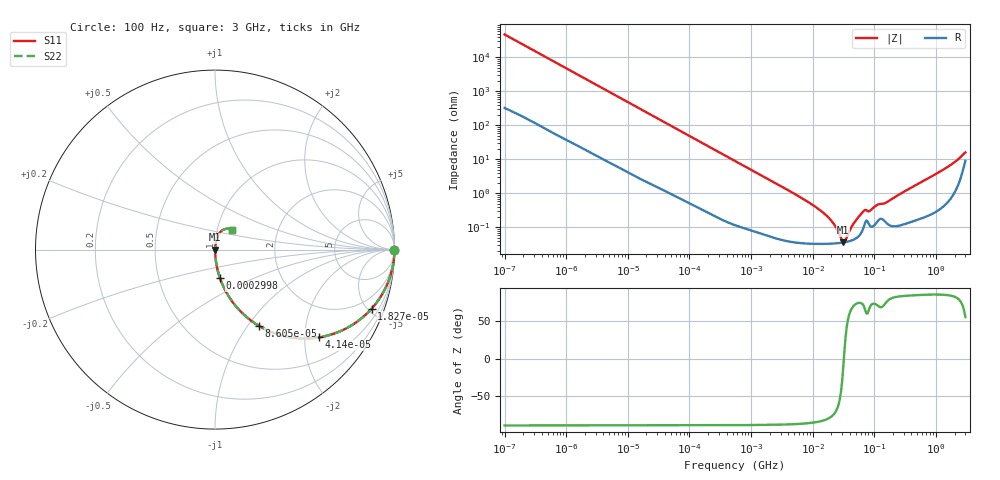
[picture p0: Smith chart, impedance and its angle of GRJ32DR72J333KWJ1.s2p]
!Murata Part Number: GRJ32DR72J333KWJ1
!These Parameters are Measured in Series Mode Connection
!Data Generated on Jun 19, 2026
!  o--ll--o
!Port1  Port2
!  o------o
!Operation Temp=25[degC], DC Bias Voltage=0[V]
!Freq. Start=100[Hz] Stop=3[GHz] 401[Steps]
# Hz S RI R 50
!Freq.(Hz) S11(Real) S11(Imag) S21(Real) S21(Imag) S12(Real) S12(Imag) S22(Real) S22(Imag)
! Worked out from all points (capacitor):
!   401 points, 100 Hz to 3 GHz, reference 50 ohm
!   read as one part in series: C = 33.7 nF near 109 Hz
!   lowest |Z| = 36.6 mohm at 31.31 MHz (marker M1)
!   series resonance near 32.03 MHz, so ESL is about 730 pH
!   S11 on the Smith chart (normalised r, x): 100 Hz: open; 18.27 kHz: 1.05, -5.30; 41.4 kHz: 1.02, -2.35; 86.05 kHz: 1.01, -1.14; 299.8 kHz: 1.00, -0.33; 3 GHz: 1.18, +0.26
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100  1 -0.00212  1.91e-05 0.00212  1.91e-05 0.00212  1 -0.00212
1788  0.9983 -0.0373  0.0017 0.0373  0.0017 0.0373  0.9983 -0.0373
6504  0.981 -0.1323  0.019 0.1323  0.019 0.1323  0.981 -0.1323
18274  0.8732 -0.3284  0.1268 0.3284  0.1268 0.3284  0.8732 -0.3284
31977  0.696 -0.4553  0.304 0.4553  0.304 0.4553  0.696 -0.4553
41399  0.5794 -0.4888  0.4206 0.4888  0.4206 0.4888  0.5794 -0.4888
86054  0.2462 -0.4257  0.7538 0.4257  0.7538 0.4257  0.2462 -0.4257
150583  0.0985 -0.2927  0.9015 0.2927  0.9015 0.2927  0.0985 -0.2927
299821  0.028 -0.1594  0.972 0.1594  0.972 0.1594  0.028 -0.1594
547723  0.0092 -0.0893  0.9908 0.0893  0.9908 0.0893  0.0092 -0.0893
9794414  0.00035 -0.00465  0.9997 0.00465  0.9997 0.00465  0.00035 -0.00465
1.950129e7  0.000333 -0.00163  0.9997 0.00163  0.9997 0.00163  0.000333 -0.00163
2.316512e7  0.000338 -0.00104  0.9997 0.00104  0.9997 0.00104  0.000338 -0.00104
3.131008e7  0.000358 -7.16e-05  0.9996 7.16e-05  0.9996 7.16e-05  0.000358 -7.16e-05
3.412477e7  0.000369 0.000204  0.9996 -0.000204  0.9996 -0.000204  0.000369 0.000204
4.612319e7  0.000436 0.00122  0.9996 -0.00122  0.9996 -0.00122  0.000436 0.00122
6.508213e7  0.000874 0.00271  0.9991 -0.00271  0.9991 -0.00271  0.000874 0.00271
8.425944e7  0.00113 0.00282  0.9989 -0.00282  0.9989 -0.00282  0.00113 0.00282
1.138854e8  0.00155 0.00439  0.9984 -0.00439  0.9984 -0.00439  0.00155 0.00439
1.751444e8  0.00119 0.00598  0.9988 -0.00598  0.9988 -0.00598  0.00119 0.00598
1.71441e9  0.0112 0.0662  0.9888 -0.0662  0.9888 -0.0662  0.0112 0.0662
3e9  0.0961 0.1088  0.9039 -0.1088  0.9039 -0.1088  0.0961 0.1088
